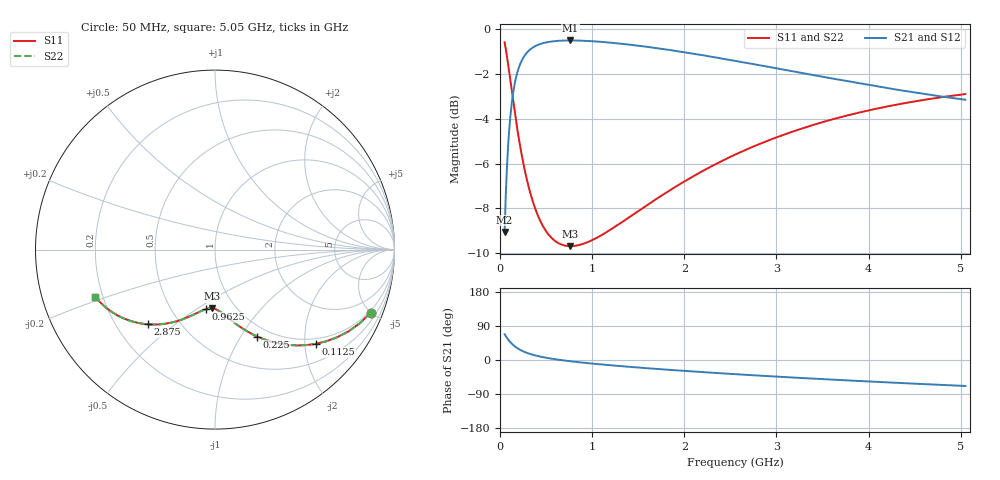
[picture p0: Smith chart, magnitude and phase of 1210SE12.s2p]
! AVX Thin Film Operation		Date: August 2001
! Description: Accu-P® Series, Thin Film, SMD, RF Capacitor
! Part Number: 12101J120FBT
! 50 MHz  -  5.05 GHz
! Serial Measurements
# mhz S db R 50
!	S11		S21		S12		S22
!	dB	Phase	dB	Phase	dB	Phase	dB	Phase
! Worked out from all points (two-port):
!   401 points, 50 MHz to 5.05 GHz, reference 50 ohm
!   highest |S21| = -0.49 dB at 762.5 MHz (marker M1); lowest = -9.1 dB at 50 MHz (marker M2)
!   |S21| within 3 dB of the highest: 122.4 MHz to end of sweep
!   lowest |S11| = -9.7 dB at 762.5 MHz (marker M3), VSWR 1.97, Z = 39 - j28.6 ohm
!   |S11| at or under -10 dB: nowhere
!   |S22| runs from -9.7 to -0.6 dB; largest |S21 - S12| = 0
!   S11 on the Smith chart (normalised r, x): 50 MHz: 0.88, -4.97; 112.5 MHz: 0.87, -2.24; 225 MHz: 0.87, -1.18; 962.5 MHz: 0.73, -0.55; 2.875 GHz: 0.33, -0.40; 5.05 GHz: 0.17, -0.18
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50  -0.57 -22.1  -9.06 67.9  -9.06 67.9  -0.57 -22.1
75  -1.19 -31.5  -6.21 58.5  -6.21 58.5  -1.19 -31.5
87.5  -1.54 -35.7  -5.25 54.3  -5.25 54.3  -1.54 -35.7
112.5  -2.29 -43.1  -3.88 46.9  -3.88 46.9  -2.29 -43.1
137.5  -3.04 -49.3  -2.98 40.7  -2.98 40.7  -3.04 -49.3
162.5  -3.77 -54.4  -2.37 35.6  -2.37 35.6  -3.77 -54.4
187.5  -4.45 -58.7  -1.93 31.2  -1.93 31.2  -4.45 -58.7
225  -5.38 -64.1  -1.49 25.9  -1.49 25.9  -5.38 -64.1
300  -6.87 -71.9  -1.00 18.1  -1.00 18.1  -6.87 -71.9
412.5  -8.34 -79.7  -0.69 10.3  -0.69 10.3  -8.34 -79.7
562.5  -9.34 -86.6  -0.54 3.3  -0.54 3.3  -9.34 -86.6
762.5  -9.70 -93.3  -0.49 -3.3  -0.49 -3.3  -9.70 -93.3
887.5  -9.62 -96.7  -0.50 -6.7  -0.50 -6.7  -9.62 -96.7
962.5  -9.50 -98.5  -0.52 -8.6  -0.52 -8.6  -9.50 -98.5
1325  -8.62 -106.5  -0.65 -16.5  -0.65 -16.5  -8.62 -106.5
1725  -7.51 -114.0  -0.85 -24.0  -0.85 -24.0  -7.51 -114.0
2125  -6.51 -120.8  -1.10 -30.8  -1.10 -30.8  -6.51 -120.8
2550  -5.61 -127.3  -1.40 -37.4  -1.40 -37.4  -5.61 -127.4
2875  -5.03 -132.1  -1.65 -42.1  -1.65 -42.1  -5.03 -132.1
3387.5  -4.29 -139.0  -2.03 -49.0  -2.03 -49.0  -4.29 -139.0
4225  -3.43 -149.3  -2.64 -59.3  -2.64 -59.3  -3.43 -149.3
5050  -2.89 -158.5  -3.15 -68.6  -3.15 -68.6  -2.89 -158.5
